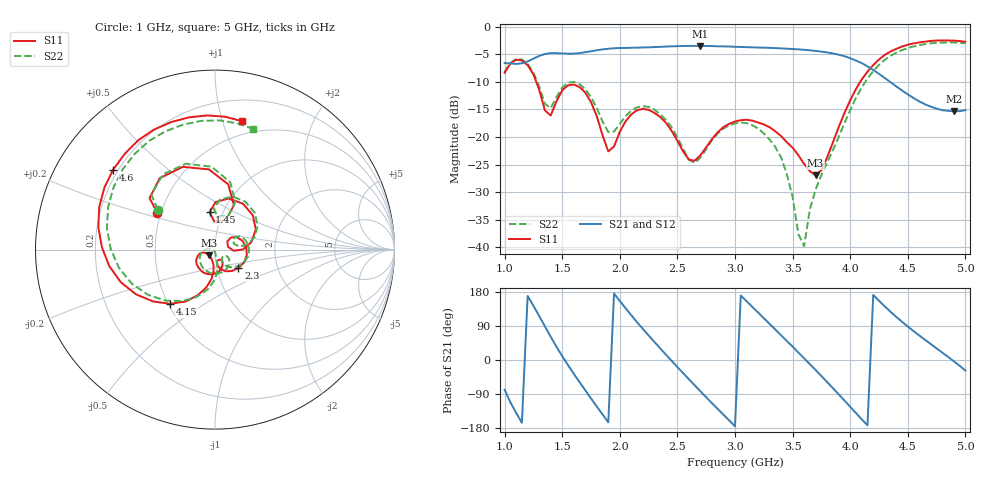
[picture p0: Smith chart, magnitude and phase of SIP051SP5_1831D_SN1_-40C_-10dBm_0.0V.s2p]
# GHz  S  dB  R  50
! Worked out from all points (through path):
!   81 points, 1 GHz to 5 GHz, reference 50 ohm
!   highest |S21| = -3.47 dB at 2.7 GHz (marker M1); lowest = -15.3 dB at 4.9 GHz (marker M2)
!   lowest |S11| = -26.9 dB at 3.7 GHz (marker M3), VSWR 1.09, Z = 46.7 - j2.92 ohm
!   |S11| at or under -10 dB: 1.275 GHz to 4.087 GHz (2.812 GHz wide, 105 % of centre)
!   |S22| runs from -39.8 to -2.8 dB; largest |S21 - S12| = 0.0037
!   S11 on the Smith chart (normalised r, x): 1 GHz: 0.48, +0.23; 1.45 GHz: 0.87, +0.38; 2.3 GHz: 1.27, -0.27; 4.15 GHz: 0.51, -0.37; 4.6 GHz: 0.18, +0.34; 5 GHz: 0.38, +1.16
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1  -8.34 147.4  -6.58 -78.4  -6.58 -78.3  -8.19 145.1
1.2  -6.97 94.3  -6.30 169.0  -6.29 168.9  -6.70 92.3
1.35  -15.15 69.4  -4.94 88.8  -4.92 88.8  -13.96 68.8
1.45  -13.53 98.2  -4.78 35.2  -4.77 35.2  -12.78 91.5
1.55  -10.62 75.0  -4.88 -13.4  -4.88 -13.4  -10.14 71.7
1.7  -11.92 26.4  -4.62 -79.8  -4.62 -79.9  -11.32 29.1
1.95  -21.72 33.6  -3.90 175.4  -3.90 175.5  -18.98 27.9
2.15  -15.14 3.6  -3.78 99.7  -3.79 100.0  -14.60 10.2
2.3  -15.61 -38.2  -3.68 47.9  -3.68 47.9  -15.01 -22.9
2.35  -16.35 -51.6  -3.64 31.0  -3.63 31.0  -15.85 -33.7
2.5  -20.69 -80.6  -3.52 -18.6  -3.51 -18.6  -20.01 -57.9
2.7  -23.30 -58.4  -3.47 -82.6  -3.46 -82.7  -23.71 -30.7
3  -17.16 -97.1  -3.63 -174.8  -3.63 -174.7  -17.53 -75.3
3.35  -18.95 -154.6  -3.87 80.4  -3.88 80.4  -21.80 -165.5
3.6  -24.86 -161.3  -4.18 4.5  -4.19 4.4  -39.78 -100.9
3.7  -26.91 -136.4  -4.39 -26.6  -4.38 -26.6  -29.50 -83.5
3.9  -18.21 -93.8  -5.06 -90.6  -5.07 -90.5  -20.02 -82.1
4.15  -8.14 -129.6  -7.18 -172.6  -7.19 -172.5  -9.40 -122.2
4.35  -4.49 -171.2  -10.06 127.3  -10.07 127.4  -5.27 -169.3
4.6  -2.84 141.9  -13.53 64.6  -13.52 64.6  -3.33 139.2
4.9  -2.51 93.2  -15.32 -3.4  -15.31 -3.4  -2.85 88.0
5  -2.72 78.1  -15.11 -27.8  -15.14 -27.9  -3.03 72.4
